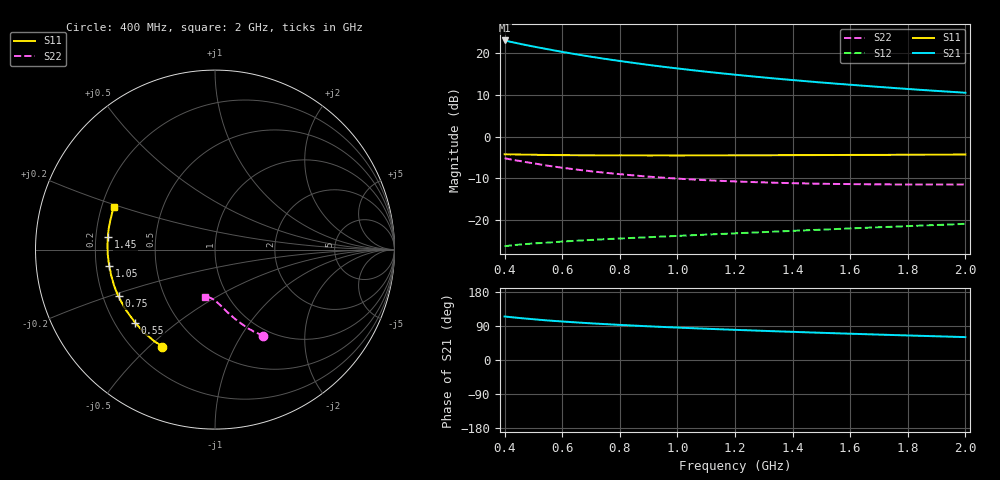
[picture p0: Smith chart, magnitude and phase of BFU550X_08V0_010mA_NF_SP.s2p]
! Filename:  P:\Prog\Test\Noise\ATS_data\Testdata_Net\BFU550X no attenuator noise\BFU550X_APG2013_44_C05_08p0V_010mA_NF_CM01_D.sf
! Date/Time: Fri 26/Jul/2013 14:37:13
! BFU550X_APG2013_44_C05_08p0V_1to10mA_NF_CM01_Bias5_R.sf
! Noise Parameter Data File
! BFU550X_APG2013_44_C05_08p0V_1to10mA_NF_CM01
! Date/time: Wed Jul 24 17:16:38 2013
! VAR V_out= 8.001000
! VAR I_out= 10.000000
! VAR V_in= 0.811500
! VAR I_in= 0.106500
! Device data file deembeded for feedlines and parallel
! Original file: \BFU550X no attenuator noise\BFU550X_APG2013_44_C05_08p0V_010mA_NF_CM01_R.sf
! Feed-files: PR005V01_100713_Feed1.s2p, PR005V01_100713_Feed2.s2p
! Parallel-file: PR005V01_100713_Par.s2p
# MHz S MA R 50
!  Freq-MHz  S11-mag  S11-arg  S21-mag  S21-arg  S12-mag  S12-arg  S22-mag  S22-arg
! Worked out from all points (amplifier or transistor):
!   37 points, 400 MHz to 2 GHz, reference 50 ohm
!   highest |S21| = 23.1 dB at 400 MHz (marker M1)
!   |S21| within 3 dB of that: start of sweep to 622.2 MHz
!   unconditionally stable (mu >= 1): 1.951 GHz to end of sweep
!   at 500 MHz: K = 0.42, MSG = 23.6 dB, |S12| = -25.6 dB
!   at 1.1 GHz: K = 0.76, MSG = 19.5 dB, |S12| = -23.5 dB
!   at 2 GHz: K = 1.00, MAG = 15.4 dB, |S12| = -20.9 dB
!   lowest NFmin = 0.78 dB at 440 MHz
!   S11 on the Smith chart (normalised r, x): 400 MHz: 0.32, -0.55; 550 MHz: 0.28, -0.36; 750 MHz: 0.26, -0.21; 1.05 GHz: 0.25, -0.07; 1.45 GHz: 0.25, +0.06; 2 GHz: 0.25, +0.19
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400  0.6155 -118.4  14.22 114.8  0.04868 43.8  0.5515 -60.7
420  0.6121 -121.2  13.71 113.2  0.04953 43.2  0.534 -62.2
440  0.6117 -124.1  13.27 111.7  0.05042 42.5  0.5194 -63.3
460  0.6092 -126.7  12.81 110.3  0.05113 41.9  0.5061 -64.7
500  0.6068 -131.8  12.03 107.5  0.0525 40.9  0.4797 -67.0
550  0.6029 -137.6  11.16 104.3  0.05372 40.1  0.4481 -69.5
600  0.5998 -142.2  10.38 101.7  0.05526 39.5  0.4244 -71.7
650  0.5996 -146.6  9.692 99.1  0.05656 39.1  0.4033 -73.8
700  0.5976 -150.6  9.084 96.8  0.0578 38.9  0.3846 -75.5
750  0.5971 -154.2  8.546 94.7  0.05905 38.8  0.3692 -77.2
800  0.5974 -157.5  8.071 92.6  0.06018 38.7  0.3551 -78.9
850  0.597 -160.7  7.638 90.7  0.06124 38.7  0.3426 -80.3
900  0.5955 -163.6  7.245 88.9  0.06233 38.9  0.3316 -81.6
950  0.5961 -166.2  6.89 87.2  0.06352 39.0  0.3224 -83.0
1050  0.5962 -171.1  6.275 84.0  0.06578 39.6  0.307 -85.3
1100  0.5967 -173.3  6.004 82.5  0.06697 39.8  0.3006 -86.4
1200  0.5979 -177.5  5.53 79.6  0.06937 40.3  0.2905 -88.5
1350  0.5997 176.8  4.937 75.6  0.07297 41.1  0.2796 -91.3
1450  0.6008 173.3  4.609 73.0  0.07554 41.7  0.2748 -93.1
1500  0.6019 171.6  4.457 71.8  0.07677 41.9  0.2725 -94.1
1750  0.6059 164.0  3.834 65.9  0.08332 43.0  0.2674 -98.2
2000  0.6114 157.2  3.361 60.4  0.09024 43.9  0.2673 -102.1
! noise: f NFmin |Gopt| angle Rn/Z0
400  0.8321  0.08297  164.8  0.087
460  0.7913  0.1295  158.3  0.071
600  0.8512  0.09332  157.4  0.0879
800  0.8541  0.1591  164.9  0.0715
1000  0.8806  0.1937  166.6  0.0669
1200  0.886  0.2238  170.3  0.0666
1400  0.9392  0.2526  174.4  0.0629
1600  0.938  0.2835  176.2  0.0612
1800  0.9814  0.3124  -177.9  0.0594
2000  1.001  0.3498  -174.7  0.0559
